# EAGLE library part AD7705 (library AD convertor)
AD7705 A-D converter (2ch) Producted by Analog Devices.Co Store Information: Digi-Key http://search.digikey.com/scripts/DkSearch/dksus.dll?Detail&name=AD7705BRUZ-ND
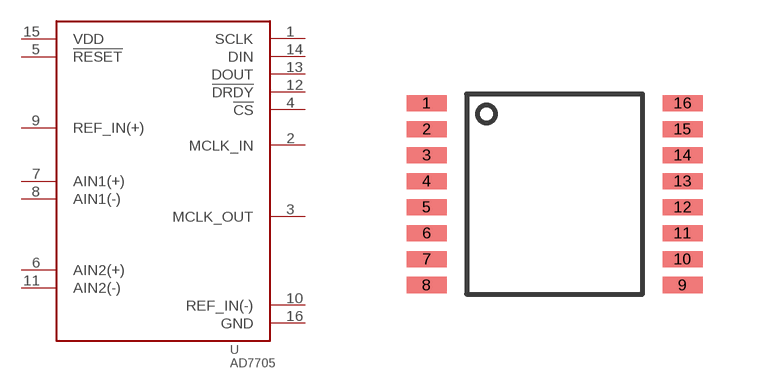
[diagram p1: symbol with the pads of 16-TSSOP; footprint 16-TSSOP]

Designator prefix U

## AD7705,16-TSSOP  [16-TSSOP]
1  SCLK
2  MCLK_IN
3  MCLK_OUT
4  !CS
5  !RESET
6  AIN2(+)
7  AIN1(+)
8  AIN1(-)
9  REF_IN(+)
10  REF_IN(-)
11  AIN2(-)
12  !DRDY
13  DOUT
14  DIN
15  VDD
16  GND

## Footprint 16-TSSOP (pad centres in mm)
4.4*5mm size , 0.65mm pitch , 16pin pacage
smd 1 x 0.4: 1 -3.2,2.275; 2 -3.2,1.625; 3 -3.2,0.975; 4 -3.2,0.325; 5 -3.2,-0.325; 6 -3.2,-0.975; 7 -3.2,-1.625; 8 -3.2,-2.275; 9 3.2,-2.275; 10 3.2,-1.625; 11 3.2,-0.975; 12 3.2,-0.325; 13 3.2,0.325; 14 3.2,0.975; 15 3.2,1.625; 16 3.2,2.275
